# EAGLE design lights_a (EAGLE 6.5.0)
REV: A; TITLE: Lights
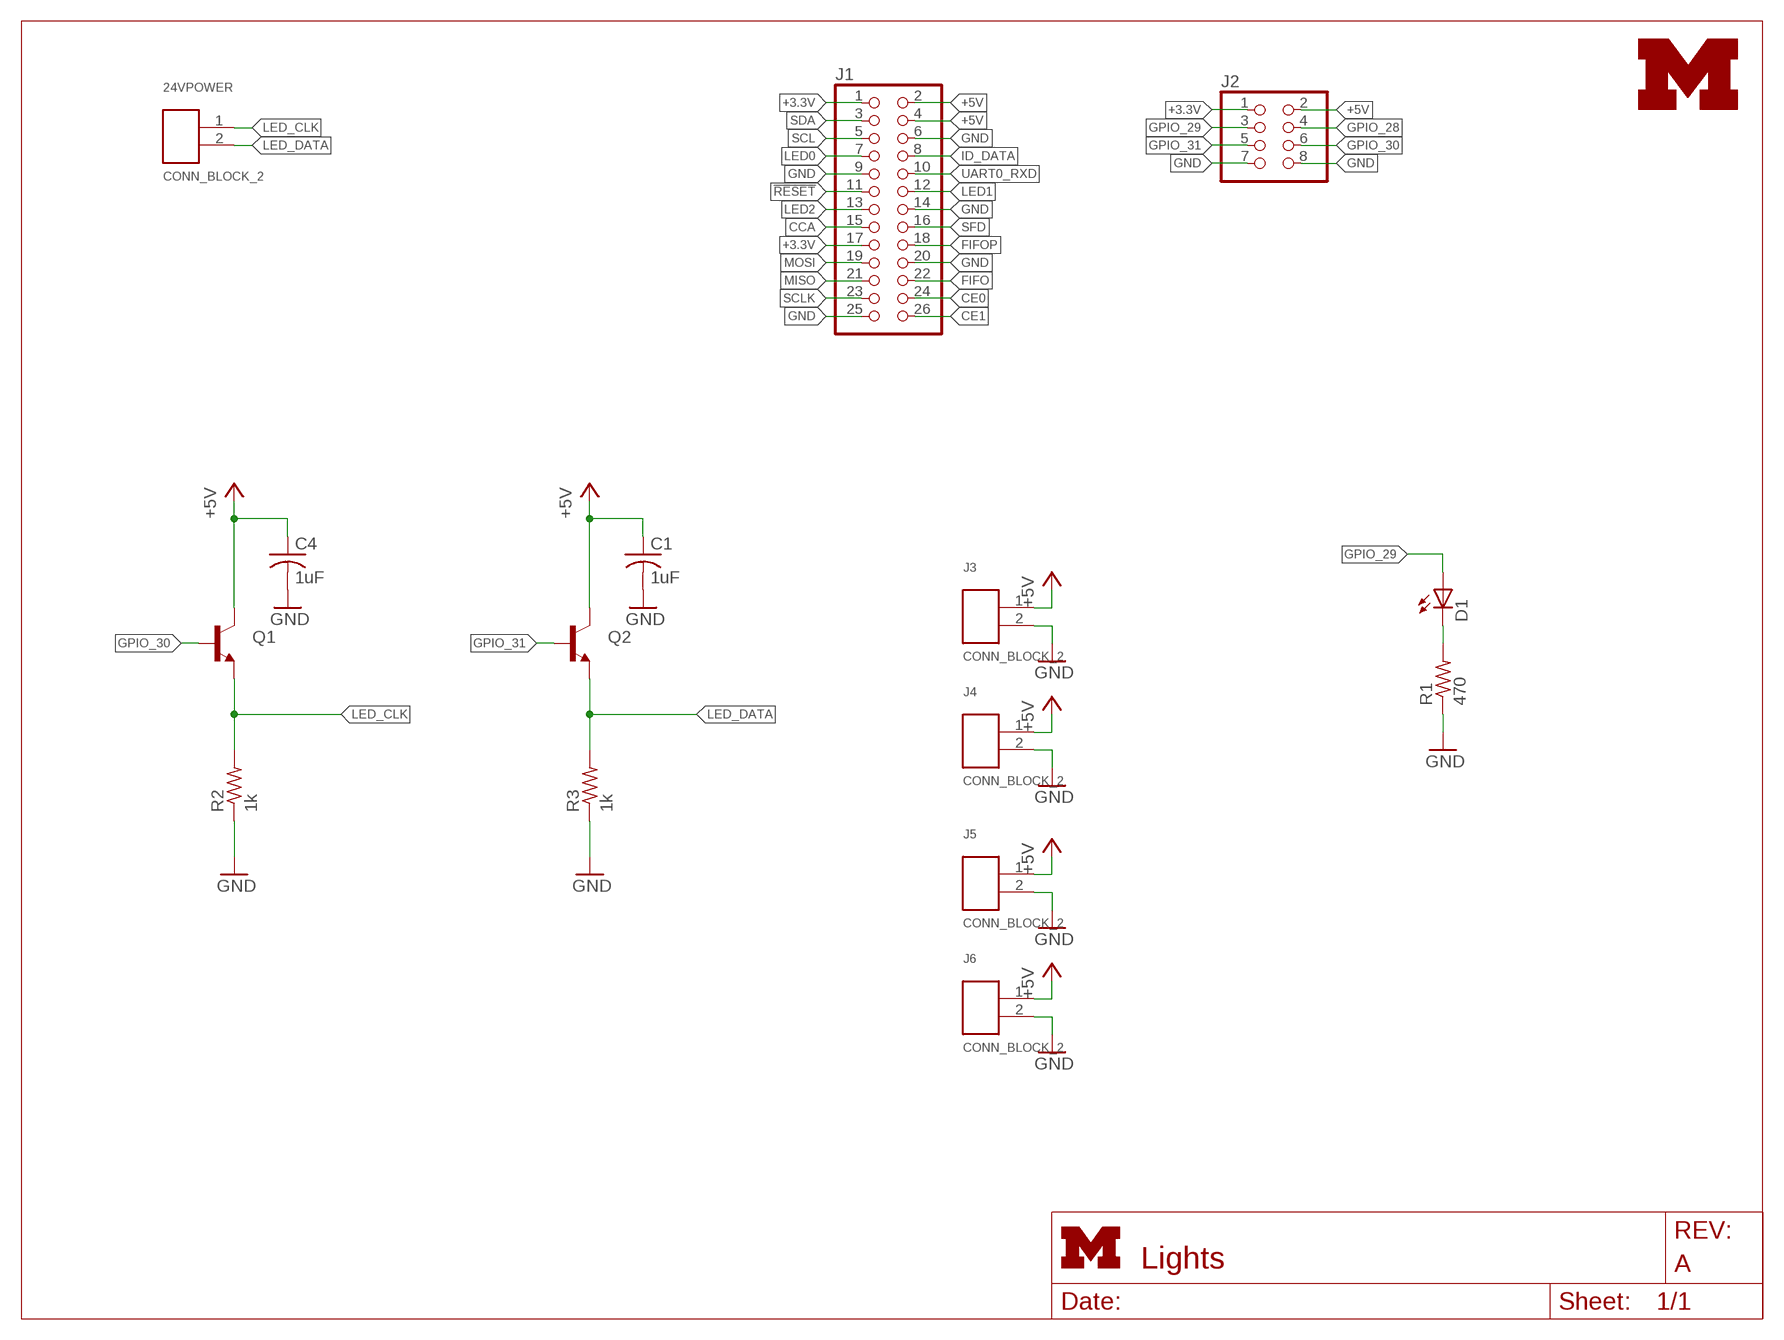
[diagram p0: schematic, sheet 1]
FRAME1 (LETTER_L): HEIGHT: 8.5in; WIDTH: 11in

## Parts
24VPOWER  CONN_BLOCK_2  [CONN_BLOCK_2]
C1  1uF  C-USC0603  [C0603]
C4  1uF  C-USC0603  [C0603]
D1  LED0603  [LED-0603]
J1  PINHD-2X13  [2X13]
J2  PINHD-2X4  [2X04]
J3  CONN_BLOCK_2  [CONN_BLOCK_2]
J4  CONN_BLOCK_2  [CONN_BLOCK_2]
J5  CONN_BLOCK_2  [CONN_BLOCK_2]
J6  CONN_BLOCK_2  [CONN_BLOCK_2]
Q1  TRANSISTOR_NPNSOT23  [SOT23]
Q2  TRANSISTOR_NPNSOT23  [SOT23]
R1  470  R-US_R0603  [R0603]
R2  1k  R-US_R0603  [R0603]
R3  1k  R-US_R0603  [R0603]
U$1  UMICH_SOLID_SMALL  [UMICH_SOLID_75MIL]

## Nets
!RESET: J1.11
+3.3V: J1.1 J1.17 J2.1
+5V: C1.1 C4.1 J1.2 J1.4 J2.2 J3.1 J4.1 J5.1 J6.1 Q1.3(C) Q2.3(C)
CCA: J1.15
CE0: J1.24
CE1: J1.26
FIFO: J1.22
FIFOP: J1.18
GND: C1.2 C4.2 J1.6 J1.9 J1.14 J1.20 J1.25 J2.7 J2.8 J3.2 J4.2 J5.2 J6.2 R1.1 R2.1 R3.1
GPIO_28: J2.4
GPIO_29: D1.A J2.3
GPIO_30: J2.6 Q1.1(B)
GPIO_31: J2.5 Q2.1(B)
ID_DATA: J1.8
LED0: J1.7
LED1: J1.12
LED2: J1.13
LED_CLK: 24VPOWER.1 Q1.2(E) R2.2
LED_DATA: 24VPOWER.2 Q2.2(E) R3.2
MISO: J1.21
MOSI: J1.19
N$1: D1.C R1.2
SCL: J1.5
SCLK: J1.23
SDA: J1.3
SFD: J1.16
UART0_RXD: J1.10

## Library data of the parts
24VPOWER J3-J6 = door-control:CONN_BLOCK_2: 2x 0.100 in screw terminal block; DIGIKEY: 277-1273-ND
C1 C4 = resistor:C-US: CAPACITOR, American symbol
D1 = SparkFun-LED:LED: LEDs; DIGIKEY: 160-1834-1-ND
J1 = pinhead:PINHD-2X13: PIN HEADER; DIGIKEY: SAM1204-13-ND
J2 = pinhead:PINHD-2X4: PIN HEADER
Q1 Q2 = door-control:TRANSISTOR_NPN: Transistor NPN BJT configuration in SOT23 package. MMBT2222 is the common NPN we use. Double check BCE configuration again layout.
R1-R3 = resistor:R-US_: RESISTOR, American symbol
U$1 = logos:UMICH_SOLID

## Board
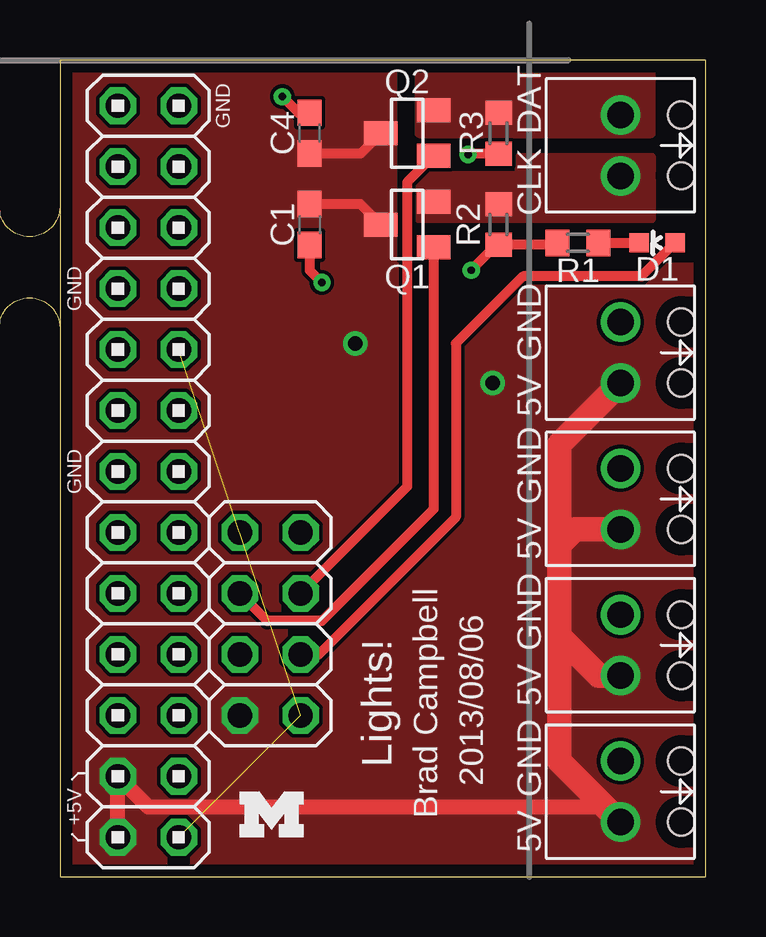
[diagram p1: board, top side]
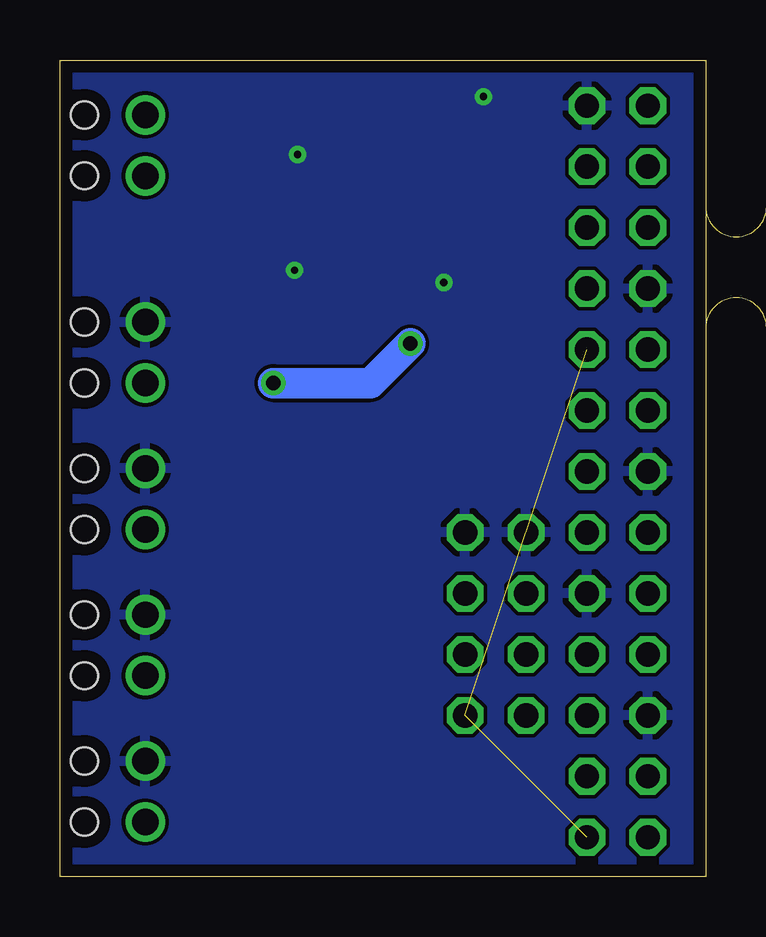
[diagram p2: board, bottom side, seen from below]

Size 26.92 x 34.04 mm. Coordinates in mm from the lower left corner, seen from the top.
Outline: 0,0 26.92,0 26.92,34.04 0,34.04 0,0
Copper layers (1*16): Top 0.0178mm / dielectric 59mil / Bottom 0.0178mm
Design rules "sunstone-2lyr_v1.0.0.3 *": minimum track width 6mil, minimum drill 14mil, track to track 6mil, track to pad 6mil, pad to pad 6mil, via to via 6mil, smd to smd 6mil, copper to edge 20mil, drill to drill 16mil, minimum pad ring 8mil, minimum via ring 8mil, stop-mask expansion 3mil, vias tented up to drill 12mil, thermal gap 10mil
Milling: 7 lines

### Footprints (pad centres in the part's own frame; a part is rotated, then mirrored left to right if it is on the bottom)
CONN_BLOCK_2 = drill 1.1: 1 -1.27,0; 2 1.27,0 | hole 1.12: -1.27,-2.54; 1.27,-2.54
C0603 = smd 1.1 x 1: 1 -0.85,0; 2 0.85,0
LED-0603 = smd 0.8 x 0.8: A 0,-0.75; C 0,0.75
2X13 = drill 1.016 octagon: 1 -15.24,-1.27; 2 -15.24,1.27; 3 -12.7,-1.27; 4 -12.7,1.27; 5 -10.16,-1.27; 6 -10.16,1.27; 7 -7.62,-1.27; 8 -7.62,1.27; 9 -5.08,-1.27; 10 -5.08,1.27; 11 -2.54,-1.27; 12 -2.54,1.27; 13 0,-1.27; 14 0,1.27; 15 2.54,-1.27; 16 2.54,1.27; 17 5.08,-1.27; 18 5.08,1.27; 19 7.62,-1.27; 20 7.62,1.27; 21 10.16,-1.27; 22 10.16,1.27; 23 12.7,-1.27; 24 12.7,1.27; 25 15.24,-1.27; 26 15.24,1.27
2X04 = drill 1.016 octagon: 1 -3.81,-1.27; 2 -3.81,1.27; 3 -1.27,-1.27; 4 -1.27,1.27; 5 1.27,-1.27; 6 1.27,1.27; 7 3.81,-1.27; 8 3.81,1.27
SOT23 = smd 1 x 1.4: 1 -0.95,-1.1; 2 0.95,-1.1; 3 0,1.1
R0603 = smd 1 x 1.1: 1 -0.85,0; 2 0.85,0

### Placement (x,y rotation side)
24VPOWER  23.37,30.48 90 top
C1  10.41,27.18 270 top
C4  10.41,30.99 90 top
D1  24.89,26.42 90 top
J1  3.68,16.89 90 top
J2  8.76,10.54 90 top
J3  23.37,15.75 90 top
J4  23.37,3.56 90 top
J5  23.37,9.65 90 top
J6  23.37,21.84 90 top
Q1  14.48,27.18 90 top
Q2  14.48,30.99 90 top
R1  21.59,26.42 0 top
R2  18.29,27.18 90 top
R3  18.29,30.99 90 top
U$1  7.49,1.65 0 top

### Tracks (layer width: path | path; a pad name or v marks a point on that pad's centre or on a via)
+3.3V  (2 unrouted)
+5V  (via drill 0.61)
  Top 0.406: Q1.3 12.53,28.03 C1.1 | Q2.3 12.53,30.14 C4.1
  Top 0.635: J4.1 22.73,2.92 3.68,2.92 J1.4 J1.2
  Top 1.016: J5.1 22.48,8.38 20.83,10.03 | 20.83,10.03 20.83,13.84 | 20.83,13.84 20.83,18.03 J6.1 | J3.1 21.46,14.48 20.83,13.84 | 20.83,10.03 20.83,4.83 J4.1
  Bottom 1.27: v18.03,20.57 13.97,20.57 v12.32,22.23
  pour Top (no thermals): 0,0 0,35.56 27.94,35.56 27.94,34.04 13.84,34.04 13.84,25.4 27.94,25.4 27.94,0
GND  (via drill 0.3)
  Top 0.406: R1.1 20.65,26.33 R2.1 18.2,26.33 v17.14,25.27 | R3.1 17.06,30.14 v17.02,30.1 | C1.2 10.41,25.27 v10.92,24.77 | C4.2 9.95,31.84 v9.27,32.51
  pour Bottom: 0,0 0,35.56 30.48,35.56 30.48,0
GPIO_29
  Top 0.406: D1.A 24.25,25.02 19.3,25.02 16.51,22.23 16.51,14.99 10.79,9.27 J2.3
GPIO_30
  Top 0.406: J2.6 8.64,10.67 10.92,10.67 15.58,15.32 Q1.1
GPIO_31
  Top 0.406: Q2.1 14.48,28.94 14.48,16.26 J2.5
LED_CLK
  Top 0.406: 15.68,28.03 Q1.2
  pour Top (no thermals): 24.64,27.43 14.99,27.43 14.99,29.21 19.18,29.21 19.18,29.97 24.64,29.97
LED_DATA
  Top 0.406: 15.68,31.84 Q2.2
  pour Top (no thermals): 24.64,33.4 14.99,33.4 14.99,30.99 24.64,30.99
N$1
  Top 0.406: R1.2 D1.C

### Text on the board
tPlace: GND | DAT | CLK | GND | GND | 5V | GND | GND | 5V | GND | 5V | Lights! | Brad Campbell | 2013/08/06 | GND | +5V | 5V
tDocu: CC2520 Edge
_tNames: Q2 | Q2 | C4 | C4 | R3 | R3 | C1 | C1 | R2 | R2 | Q1 | Q1 | R1 | R1 | D1 | D1

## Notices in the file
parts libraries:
SparkFun-LED: Licensing: CC v3.0 Share-Alike You are welcome to use this library for commercial purposes.
